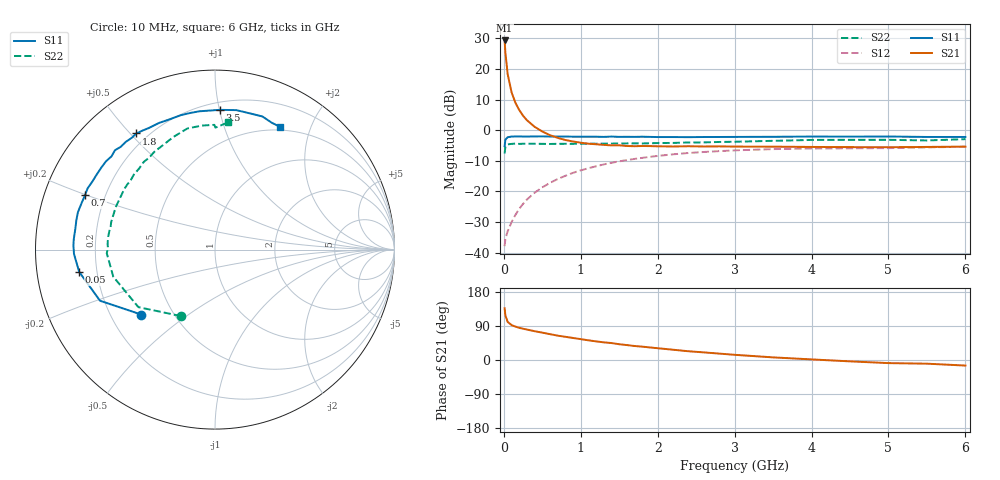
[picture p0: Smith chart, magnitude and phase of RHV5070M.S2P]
! SIEMENS Small Signal Semiconductors
! BFR106
! Si NPN RF Bipolar Junction Transistor in SOT23
! VCE = 0.5 V  IC = 70 mA
! Common Emitter S-Parameters:  August  1996
# GHz  S  MA  R  50
!  f  S11  S21  S12  S22
! GHz  MAG  ANG  MAG  ANG  MAG  ANG  MAG  ANG
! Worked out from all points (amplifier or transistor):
!   36 points, 10 MHz to 6 GHz, reference 50 ohm
!   highest |S21| = 29.3 dB at 10 MHz (marker M1)
!   |S21| within 3 dB of that: start of sweep to 17.62 MHz
!   unconditionally stable (mu >= 1): 45.14 MHz to end of sweep
!   at 250 MHz: K = 1.63, MAG = 9.8 dB, |S12| = -24.1 dB
!   at 1.4 GHz: K = 1.29, MAG = -0.4 dB, |S12| = -10.7 dB
!   at 6 GHz: K = 1.04, MAG = -1.1 dB, |S12| = -5.4 dB
!   S11 on the Smith chart (normalised r, x): 10 MHz: 0.33, -0.34; 50 MHz: 0.13, -0.08; 700 MHz: 0.13, +0.20; 1.8 GHz: 0.16, +0.52; 3.5 GHz: 0.25, +1.00; 6 GHz: 0.46, +1.56
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0.01  0.5473 -138.6  29.27 136.7  0.0127 49.3  0.4163 -117.2
0.02  0.7009 -156.0  18.6 117.6  0.0168 40.2  0.5339 -143.1
0.05  0.7665 -170.6  8.193 100.5  0.0223 42.3  0.5865 -165.1
0.1  0.786 -178.2  4.176 92.2  0.0313 53.3  0.5961 -174.8
0.15  0.789 178.5  2.81 88.1  0.0411 60.2  0.6034 -178.1
0.2  0.789 175.9  2.135 85.0  0.0518 64.1  0.5964 179.3
0.25  0.7873 173.6  1.719 82.5  0.0624 66.2  0.5993 177.0
0.3  0.7866 171.8  1.456 80.4  0.0735 67.1  0.5991 175.6
0.4  0.7897 167.9  1.136 76.0  0.095 67.8  0.5992 172.7
0.5  0.7916 164.7  0.95 72.2  0.1163 67.2  0.5974 170.0
0.6  0.7871 160.6  0.828 68.2  0.1376 66.0  0.5948 167.8
0.7  0.7851 157.3  0.749 64.3  0.1589 64.7  0.598 165.6
0.8  0.7876 154.3  0.69 61.2  0.1794 62.8  0.5987 163.1
1.1  0.781 144.3  0.601 51.9  0.239 57.0  0.6016 156.6
1.8  0.7816 124.1  0.551 35.2  0.3528 42.2  0.6069 141.3
2.2  0.7716 113.9  0.541 27.1  0.403 34.1  0.6186 133.1
2.8  0.7738 100.1  0.543 16.9  0.4543 23.0  0.6416 121.7
3.5  0.7791 88.0  0.537 6.9  0.4902 12.0  0.6692 110.2
4.5  0.7835 75.4  0.528 -3.6  0.505 -0.7  0.6949 96.1
5  0.7874 70.4  0.526 -8.2  0.5085 -5.5  0.695 90.3
5.5  0.7742 65.8  0.532 -9.7  0.523 -7.8  0.6793 89.8
6  0.7741 62.2  0.538 -14.7  0.536 -13.5  0.7129 84.1
